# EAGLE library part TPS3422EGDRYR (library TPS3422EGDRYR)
Single Channel Push Button Controller with Configurable Delay and Reset Pulse Source: Datasheet
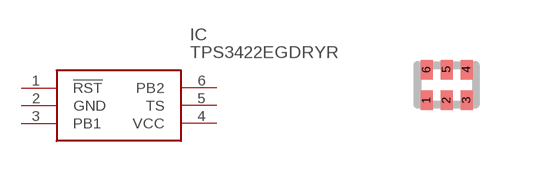
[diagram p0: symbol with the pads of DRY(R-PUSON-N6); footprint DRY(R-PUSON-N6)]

Designator prefix IC

## TPS3422EGDRYR (Arrow_Part_Number: TPS3422EGDRYR; Arrow_Price-Stock: https://www.arrow.com/en/products/tps3422egdryr/texas-instruments?utm_currency=USD&region=nac; Description: Single Channel Push Button Controller with Configurable Delay and Reset Pulse; Height: mm; Manufacturer_Name: Texas Instruments; Manufacturer_Part_Number: TPS3422EGDRYR; Mouser_Part_Number: 595-TPS3422EGDRYR; Mouser_Price-Stock: https://www.mouser.co.uk/ProductDetail/Texas-Instruments/TPS3422EGDRYR?qs=%252BrH4t%252BeVZ2OD4BsbWUMJIA%3D%3D)  [DRY(R-PUSON-N6)]
1  !RST
2  GND
3  PB1
4  VCC
5  TS
6  PB2

## Footprint DRY(R-PUSON-N6) (pad centres in mm)
DRY (R-PUSON-N6)
smd 0.3 x 0.49: 1 -0.5,-0.385; 2 0,-0.385; 3 0.5,-0.385; 4 0.5,0.385; 5 0,0.385; 6 -0.5,0.385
